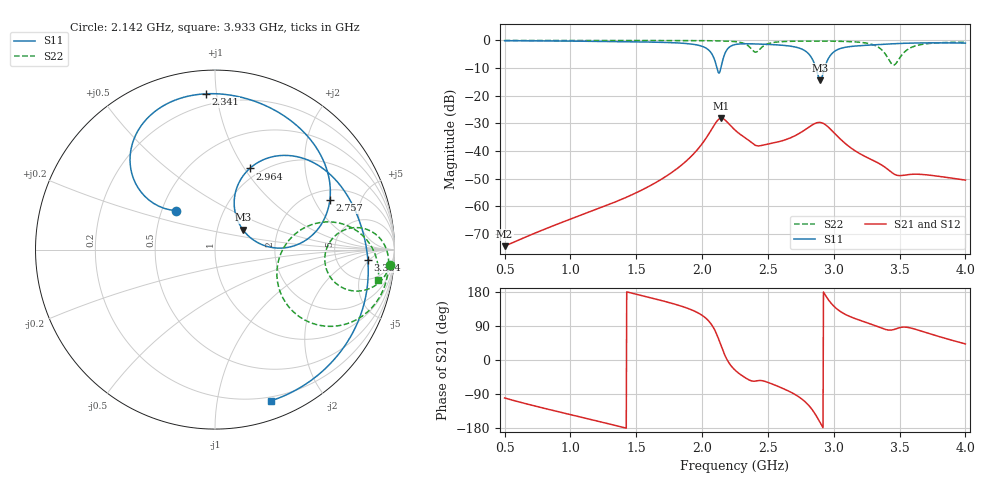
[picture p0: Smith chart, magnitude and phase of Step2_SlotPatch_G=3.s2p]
! TOUCHSTONE file generated by CST MICROWAVE STUDIO
! Date and time: Mon May 18 02:25:55 2020
! Project name: DualBand_DualMode_Antenna_FD_SteppedDesign.cst
! Parameters = {FPL=20; FPW=20; L=50; ST=10; SW=30; W=52; WF=7; ext=10; gap=1; inset=13}
! Header version: 2015
! Port assignment regex: !\s*Touchstone port\s*([0-9]+)\s*=\s*CST MWS port\s*([0-9]+)\s*\(\"(.*)\"\)(\s*mode\s*([0-9]+))?.*
! Touchstone port assignment:
! Touchstone port 1 = CST MWS port 1 ("")
! Touchstone port 2 = CST MWS port 2 ("")
# GHz S MA R 50
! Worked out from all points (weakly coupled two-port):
!   1006 points, 500 MHz to 4 GHz, reference 50 ohm
!   highest |S21| = -28.14 dB at 2.145 GHz (marker M1); lowest = -74.4 dB at 500 MHz (marker M2)
!   lowest |S11| = -14.4 dB at 2.897 GHz (marker M3), VSWR 1.47, Z = 66.4 + j15.3 ohm
!   |S11| at or under -10 dB: 2.113 GHz to 2.143 GHz (29.48 MHz wide, 1.39 % of centre); 2.865 GHz to 2.93 GHz (65.53 MHz wide, 2.26 % of centre)
!   |S22| runs from -8.9 to 0.0 dB; largest |S21 - S12| = 3.2e-05
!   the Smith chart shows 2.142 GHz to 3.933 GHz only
!   S11 on the Smith chart (normalised r, x): 2.142 GHz: 0.59, +0.28; 2.341 GHz: 0.13, +0.93; 2.757 GHz: 2.50, +2.68; 2.964 GHz: 0.89, +1.06; 3.384 GHz: 11, -4; 3.933 GHz: 0.16, -1.43
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0.5  0.9887 -61.5  0.0001903 -100.2  0.0001903 -100.2  0.9976 42.8
0.7905  0.9819 -97.0  0.0003748 -126.6  0.0003748 -126.7  0.9981 25.7
1.0845  0.9673 -133.1  0.0006993 -151.2  0.0006981 -151.0  0.9979 16.3
1.669  0.9259 155.1  0.002873 159.0  0.002874 159.1  0.9956 4.8
1.9875  0.7997 106.4  0.01236 120.7  0.01236 120.7  0.9906 -1.0
2.089  0.4847 82.9  0.02868 83.7  0.02867 83.7  0.985 -3.4
2.1415  0.3078 135.1  0.03908 40.2  0.03905 40.2  0.9788 -4.9
2.145  0.3346 138.6  0.03917 36.9  0.03914 36.9  0.9783 -5.1
2.187  0.6677 135.0  0.03406 2.5  0.03405 2.5  0.972 -6.5
2.25  0.8404 113.2  0.02393 -26.6  0.02393 -26.6  0.9521 -9.5
2.341  0.8696 93.4  0.01643 -49.5  0.01643 -49.6  0.8285 -16.2
2.46  0.8547 74.3  0.01274 -54.9  0.01274 -54.9  0.7734 9.0
2.7575  0.6969 23.3  0.0222 -102.9  0.02219 -102.9  0.9707 -4.4
2.8345  0.4728 4.0  0.02941 -130.2  0.0294 -130.2  0.9721 -6.7
2.8975  0.1908 35.6  0.03281 -165.5  0.03281 -165.5  0.9714 -8.5
2.964  0.4917 66.8  0.02636 156.9  0.02636 156.9  0.9696 -10.5
3.1285  0.7761 30.0  0.01147 113.8  0.01147 113.8  0.9502 -17.0
3.384  0.8533 -3.8  0.005198 81.6  0.005191 81.5  0.6007 -38.5
3.419  0.8623 -8.0  0.004488 79.0  0.004482 78.9  0.4471 -34.2
3.545  0.8882 -23.4  0.003686 86.8  0.003684 86.8  0.6397 14.0
3.9335  0.8985 -69.6  0.00314 48.7  0.00314 48.7  0.9256 -10.5
4  0.8925 -77.3  0.00298 42.4  0.00298 42.4  0.9286 -13.4
